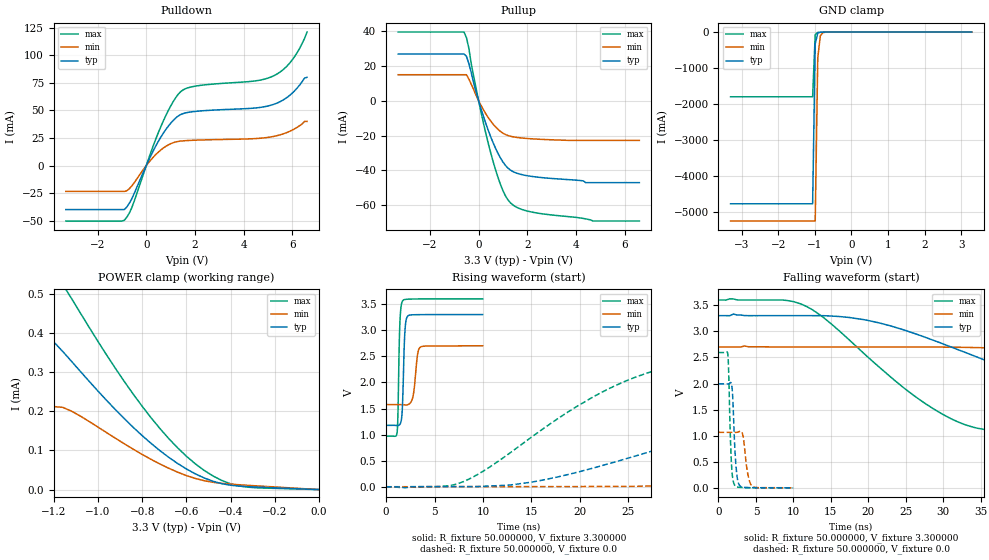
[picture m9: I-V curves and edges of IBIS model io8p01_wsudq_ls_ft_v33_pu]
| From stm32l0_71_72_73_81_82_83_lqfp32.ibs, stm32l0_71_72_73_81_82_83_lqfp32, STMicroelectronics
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|   Model io8p01_wsudq_ls_ft_v33_pu
[Model]  io8p01_wsudq_ls_ft_v33_pu
Model_type I/O
Polarity   Non-Inverting
Enable   Active-Low
Vinl =   0.990000V
Vinh =   2.310000V
Vmeas =  1.650000V
Cref =   50.000000pF
Rref =   100.000000M
Vref =   0.0V
C_comp   2.653200pF   2.620200pF   2.695100pF
[Temperature Range]   25.000000   0.125000k   -40.000000
[Pullup Reference]   3.300000V   2.700000V   3.600000V
[Pulldown Reference]   0.0V   0.0V   0.0V
[POWER Clamp Reference]   3.300000V   2.700000V   3.600000V
[GND Clamp Reference]   0.0V   0.0V   0.0V
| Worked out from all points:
|   slope of the pulldown table from 0 to 0.495 V, typ, clamps not added: 22.6 ohm
|   slope of the pullup table from 0 to 0.495 V, typ, clamps not added: 23.9 ohm
|   GND clamp passes 1 mA (typ) near -0.64 V on its own axis
|   POWER clamp passes 1 mA (typ) near -2.97 V on its own axis
|   rising waveform, R_fixture 50.000000, V_fixture 3.300000: 20-80 % time 213ps typ, 362ps min, 177ps max; typ from 1.18 V to 3.3 V
|   rising waveform, R_fixture 50.000000, V_fixture 0.0: 20-80 % time 27ns typ, 59.5ns min, 13.6ns max; typ from 0.001 V to 1.99 V
|   falling waveform, R_fixture 50.000000, V_fixture 3.300000: 20-80 % time 24.2ns typ, 53.5ns min, 13.3ns max; typ from 3.3 V to 1.18 V
|   falling waveform, R_fixture 50.000000, V_fixture 0.0: 20-80 % time 403ps typ, 569ps min, 325ps max; typ from 1.99 V to 0.001 V
[Pulldown]
|Voltage   I(typ)   I(min)   I(max)
-3.3V     -39.83mA   -23.37mA   -50.2mA
-900mV    -39.83mA   -23.37mA   -49.52mA
-600mV    -30.28mA   -18.59mA   -38.45mA
500mV     22.11mA    12.28mA    30.1mA
1V        38.33mA    19.81mA    53.88mA
1.4V      46.1mA     22.18mA    66.72mA
2V        49.07mA    23.01mA    71.93mA
4.4V      52.05mA    24.38mA    76.53mA
5.2V      55.25mA    26.3mA     81.02mA
6V        65.78mA    32.24mA    95.96mA
6.3V      73.08mA    36.2mA     106.4mA
6.6V      80mA       40mA       121mA
[Pullup]
|Voltage   I(typ)   I(min)   I(max)
-3.3V     26.68mA    14.83mA    39.29mA
-600mV    26.68mA    14.83mA    39.29mA
-500mV    25.41mA    14.83mA    36.13mA
-400mV    21.18mA    12.36mA    30.01mA
-300mV    15.95mA    9.33mA     20.96mA
100mV     -4.685mA   -2.744mA   -6.646mA
600mV     -24.28mA   -13.56mA   -35.12mA
1V        -35.19mA   -18.68mA   -51.62mA
1.4V      -40.59mA   -20.71mA   -59.71mA
2.2V      -43.48mA   -21.92mA   -63.91mA
4.7V      -47mA      -22.8mA    -69mA
6.6V      -47mA      -22.8mA    -69mA
[GND_clamp]
|Voltage   I(typ)   I(min)   I(max)
-3.3V     -4.766A    -5.244A    -1.797A
-1.06V    -4.766A    -5.244A    -1.797A
-990mV    -326.7mA   -5.244A    -68.05mA
-920mV    -29.09mA   -722.2mA   -11.16mA
-850mV    -6.797mA   -104.4mA   -6.682mA
-780mV    -3.554mA   -17.44mA   -4.265mA
-500mV    -58.08uA   -169.3uA   -34.1uA
3.28V     0A         0A         0A
[POWER_clamp]
|Voltage   I(typ)   I(min)   I(max)
-3.28V    3.05A      226.6uA    3.724A
-2.96V    694.9uA    211.8uA    3.724A
-2.92V    479.6uA    211.8uA    509.1mA
-2.88V    432uA      211.8uA    70.08mA
-2.76V    412.8uA    211.8uA    794.1uA
-1.32V    411.6uA    211.8uA    593.3uA
-1.24V    395.5uA    211.8uA    578.2uA
-1.12V    327.2uA    200.2uA    487.6uA
-800mV    137.6uA    89.62uA    212.3uA
-560mV    40.27uA    28.42uA    65.81uA
-360mV    8.799uA    12.27uA    9.112uA
0V        0A         0A         0A
[Ramp]
| variable   typ   min   max
dV/dt_r  1.19492/26.97638n   0.63587/59.52749n   1.55547/13.56604n
dV/dt_f  1.27344/24.19715n   0.66972/53.47808n   1.57816/13.29199n
R_load = 50.000000
[Rising Waveform]
R_fixture= 50.000000
V_fixture= 3.300000
V_fixture_min= 2.700000
V_fixture_max= 3.600000
|time   V(typ)   V(min)   V(max)
0s        1.178V     1.575V     969.7mV
1.141ns   1.174V     1.576V     1.058V
1.221ns   1.174V     1.576V     1.44V
1.421ns   1.198V     1.575V     3.153V
1.702ns   1.641V     1.573V     3.562V
1.922ns   2.932V     1.57V      3.588V
2.222ns   3.269V     1.573V     3.594V
2.783ns   3.295V     1.742V     3.597V
3.483ns   3.298V     2.668V     3.599V
9.97ns    3.3V       2.7V       3.6V
[Rising Waveform]
R_fixture= 50.000000
V_fixture= 0.0
V_fixture_min= 0.0
V_fixture_max= 0.0
|time   V(typ)   V(min)   V(max)
0s        1.061mV    1.817mV    656.1uV
7.508ns   3.314mV    4.291mV    67.84mV
15.02ns   89.71mV    4.323mV    952.9mV
24.52ns   524.3mV    8.386mV    2.009V
30.53ns   852.7mV    30.02mV    2.355V
38.54ns   1.236V     81.65mV    2.519V
54.55ns   1.713V     257.7mV    2.583V
76.08ns   1.928V     535.5mV    2.592V
136.6ns   1.992V     968.1mV    2.593V
249.2ns   1.993V     1.064V     2.593V
[Falling Waveform]
R_fixture= 50.000000
V_fixture= 3.300000
V_fixture_min= 2.700000
V_fixture_max= 3.600000
|time   V(typ)   V(min)   V(max)
0s        3.3V       2.7V       3.6V
11.51ns   3.3V       2.7V       3.491V
19.52ns   3.22V      2.7V       2.56V
28.53ns   2.836V     2.699V     1.529V
33.03ns   2.589V     2.692V     1.204V
38.54ns   2.277V     2.67V      1.066V
55.56ns   1.485V     2.522V     988.6mV
76.08ns   1.262V     2.24V      974mV
131.1ns   1.185V     1.707V     969.9mV
249.2ns   1.178V     1.575V     969.7mV
[Falling Waveform]
R_fixture= 50.000000
V_fixture= 0.0
V_fixture_min= 0.0
V_fixture_max= 0.0
|time   V(typ)   V(min)   V(max)
0s        1.993V     1.064V     2.593V
1.241ns   1.992V     1.064V     2.561V
1.341ns   1.993V     1.064V     2.297V
1.722ns   1.999V     1.064V     488.1mV
1.902ns   1.733V     1.064V     182.2mV
2.142ns   874.8mV    1.064V     54.84mV
2.503ns   194.1mV    1.066V     16.7mV
2.923ns   30.42mV    1.089V     9.1mV
4.424ns   4.244mV    42.33mV    2.25mV
9.97ns    1.061mV    1.817mV    656.1uV
